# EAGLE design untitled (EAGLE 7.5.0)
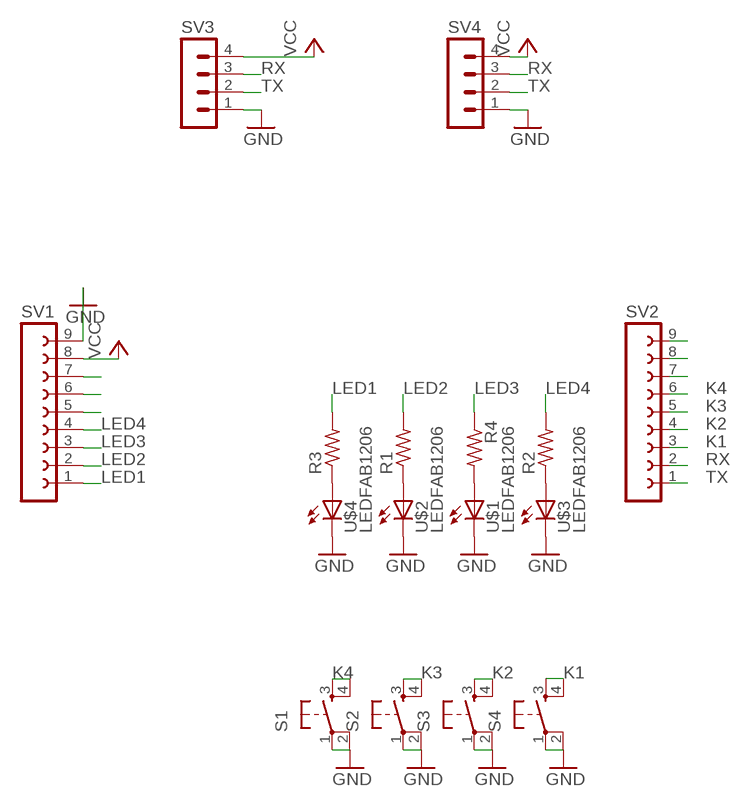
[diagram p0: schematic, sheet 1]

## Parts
R1  RES-US1206FAB  [R1206FAB]
R2  RES-US1206FAB  [R1206FAB]
R3  RES-US1206FAB  [R1206FAB]
R4  RES-US1206FAB  [R1206FAB]
S1  6MM_SWITCH6MM_SWITCH  [6MM_SWITCH]
S2  6MM_SWITCH6MM_SWITCH  [6MM_SWITCH]
S3  6MM_SWITCH6MM_SWITCH  [6MM_SWITCH]
S4  6MM_SWITCH6MM_SWITCH  [6MM_SWITCH]
SV1  FE09-1  [FE09]
SV2  FE09-1  [FE09]
SV3  MA04-1  [MA04-1]
SV4  MA04-1  [MA04-1]
U$1  LEDFAB1206  [LED1206FAB]
U$2  LEDFAB1206  [LED1206FAB]
U$3  LEDFAB1206  [LED1206FAB]
U$4  LEDFAB1206  [LED1206FAB]

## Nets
GND: S1.1(P) S1.2(P1) S2.1(P) S2.2(P1) S3.1(P) S3.2(P1) S4.1(P) S4.2(P1) SV1.9 SV3.1 SV4.1 U$1.2(C) U$2.2(C) U$3.2(C) U$4.2(C)
K1: S4.3(S) S4.4(S1) SV2.3
K2: S3.3(S) S3.4(S1) SV2.4
K3: S2.3(S) S2.4(S1) SV2.5
K4: S1.3(S) S1.4(S1) SV2.6
LED1: R3.2 SV1.1
LED2: R1.2 SV1.2
LED3: R4.1 SV1.3
LED4: R2.2 SV1.4
N$1: SV2.8
N$2: SV2.9
N$3: SV2.7
N$12: SV1.7
N$13: SV1.6
N$18: R3.1 U$4.1(A)
N$19: R1.1 U$2.1(A)
N$20: R4.2 U$1.1(A)
N$21: R2.1 U$3.1(A)
N$22: SV1.5
RX: SV2.2 SV3.3 SV4.3
TX: SV2.1 SV3.2 SV4.2
VCC: SV1.8 SV3.4 SV4.4

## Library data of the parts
R1-R4 = fab:RES-US: Resistor (US Symbol)
S1-S4 = fab:6MM_SWITCH: OMRON SWITCH
SV1 SV2 = con-lsta:FE09-1: FEMALE HEADER; OC_FARNELL: unknown; OC_NEWARK: unknown
SV3 SV4 = con-lstb:MA04-1: PIN HEADER; OC_FARNELL: unknown; OC_NEWARK: unknown
U$1-U$4 = fab:LED: LED

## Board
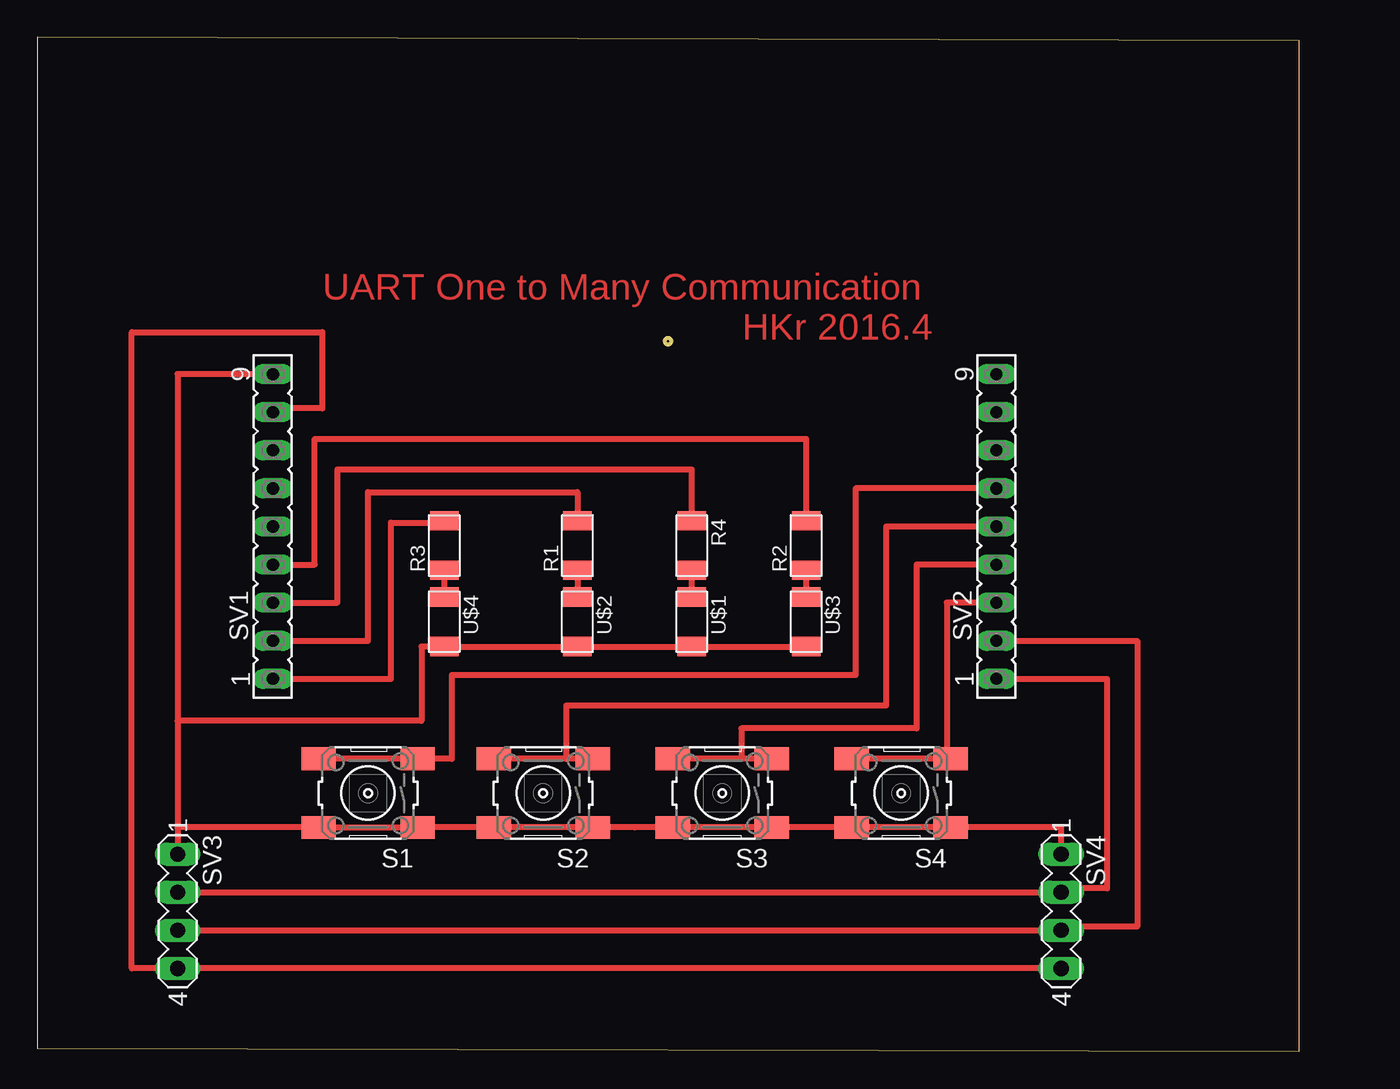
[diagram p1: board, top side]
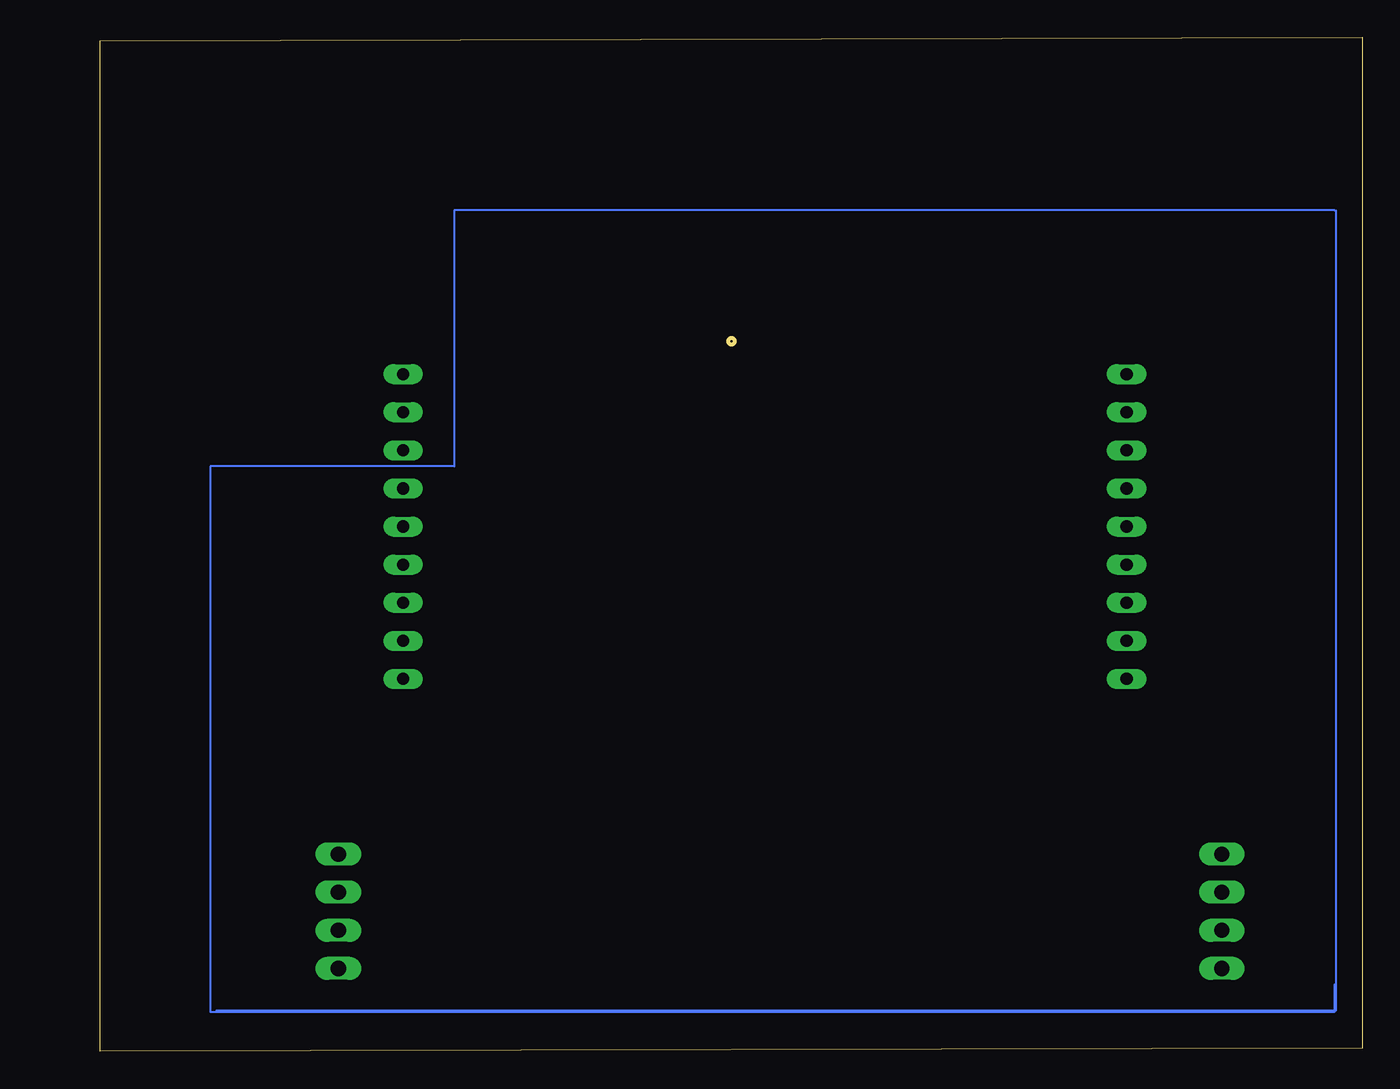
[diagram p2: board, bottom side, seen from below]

Size 84.15 x 67.6 mm. Coordinates in mm from the lower left corner, seen from the top.
Outline: 0,0.2 84.15,0 84.15,67.4 0,67.61 0,0.2
Copper layers (1*16): Top 0.035mm / dielectric 1.5mm / Bottom 0.035mm
Design rules "default": minimum track width 10mil, minimum drill 24mil, track to track 8mil, track to pad 8mil, pad to pad 8mil, via to via 8mil, smd to smd 8mil, copper to edge 40mil, drill to drill 8mil, minimum pad ring 10mil, minimum via ring 8mil, stop-mask expansion 4mil, vias tented up to drill 0mil, thermal gap 10mil
Milling: area 41.9,47.1 to 42.3,47.5

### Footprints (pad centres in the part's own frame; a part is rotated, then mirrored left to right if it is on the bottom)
R1206FAB = smd 1.27 x 1.905: 1 -1.651,0; 2 1.651,0
6MM_SWITCH = smd 2.286 x 1.524: 1 -3.302,2.286; 2 3.302,2.286; 3 -3.302,-2.286; 4 3.302,-2.286
FE09 = drill 0.813 long: 1 -10.16,0; 2 -7.62,0; 3 -5.08,0; 4 -2.54,0; 5 0,0; 6 2.54,0; 7 5.08,0; 8 7.62,0; 9 10.16,0
MA04-1 = drill 1.016 long: 1 -3.81,0; 2 -1.27,0; 3 1.27,0; 4 3.81,0
LED1206FAB = smd 1.27 x 1.905: 1 -1.651,0; 2 1.651,0

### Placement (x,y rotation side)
R1  36.02,33.73 90 top
R2  51.26,33.73 90 top
R3  27.13,33.73 90 top
R4  43.64,33.73 270 top
S1  22.05,17.22 180 top
S2  33.73,17.22 180 top
S3  45.67,17.22 180 top
S4  57.61,17.22 180 top
SV1  15.7,35 90 top
SV2  63.96,35 90 top
SV3  9.35,9.35 270 top
SV4  68.28,9.35 270 top
U$1  43.64,28.65 270 top
U$2  36.02,28.65 270 top
U$3  51.26,28.65 270 top
U$4  27.13,28.65 270 top

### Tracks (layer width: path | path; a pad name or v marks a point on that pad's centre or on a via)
GND
  Top 0.406: U$3.2 U$1.2 U$2.2 U$4.2 25.6,27 25.6,22.05 9.35,22.05 | S4.1 S4.2 | S4.1 S3.1 S3.2 | S3.2 39.83,14.94 | S3.2 S2.1 S2.2 S1.1 S1.2 9.35,14.94 SV3.1 9.35,22.05 | SV1.9 9.35,45.16 9.35,22.05 | SV4.1 68.28,14.94 S4.1
K1
  Top 0.406: SV2.3 60.66,29.92 60.66,19.51 S4.3 S4.4
K2
  Top 0.406: SV2.4 58.62,32.46 58.62,21.54 46.94,21.54 46.94,19.51 | S3.3 46.94,19.51 | 46.94,19.51 S3.4
K3
  Top 0.406: SV2.5 56.59,35 56.59,23.06 35.26,23.06 35.26,19.51 | S2.3 35.26,19.51 | 35.26,19.51 S2.4
K4
  Top 0.406: S1.4 S1.3 27.64,19.51 27.64,25.1 54.56,25.1 54.56,37.54 SV2.6
LED1
  Top 0.406: SV1.1 23.57,24.84 23.57,35.26 27.13,35.26 R3.2
LED2
  Top 0.406: SV1.2 22.05,27.38 22.05,37.29 36.02,37.29 R1.2
LED3
  Top 0.406: SV1.3 20.02,29.92 20.02,38.81 43.64,38.81 R4.1
LED4
  Top 0.406: SV1.4 18.49,32.46 18.49,40.84 51.26,40.84 R2.2
N$4
  Bottom 0.127: 76.4,2.74 1.73,2.74 1.73,56.08
N$5
  Bottom 0.127: 1.83,56.08 60.55,56.08 60.55,39.01 76.81,39.01 76.81,2.64 1.83,2.64 1.83,4.47
N$18
  Top 0.406: R3.1 U$4.1
N$19
  Top 0.406: R1.1 U$2.1
N$20
  Top 0.406: R4.2 U$1.1
N$21
  Top 0.406: R2.1 U$3.1
RX
  Top 0.406: SV2.2 73.36,27.38 73.36,8.33 68.28,8.33 SV4.3 SV3.3
TX
  Top 0.406: SV2.1 71.32,24.84 71.32,10.87 68.28,10.87 SV4.2 SV3.2
VCC
  Top 0.406: SV1.8 15.7,42.88 19,42.88 19,47.96 6.3,47.96 6.3,5.54 SV3.4 SV4.4

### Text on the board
Top: UART One to Many Communication / HKr 2016.4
